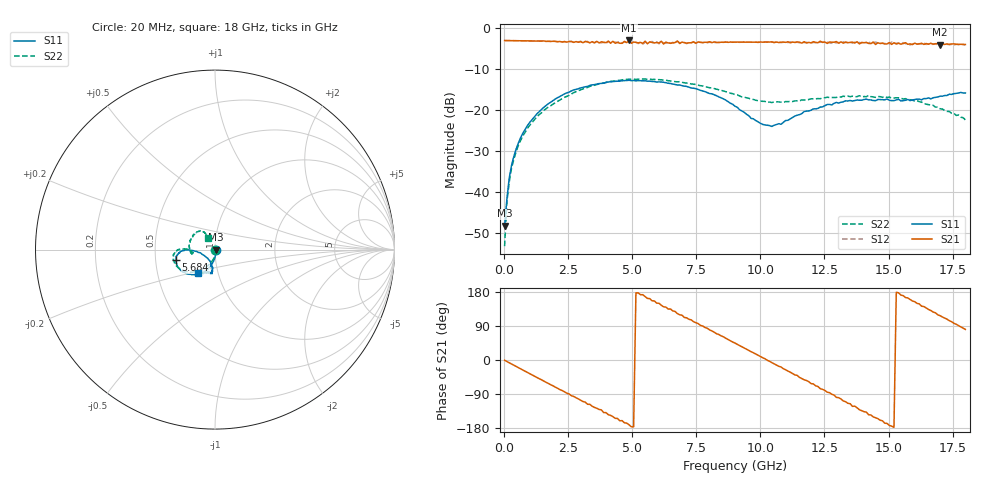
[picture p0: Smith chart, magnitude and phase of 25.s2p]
!Agilent Technologies,N5230A,US43500223,A.07.50.48
!Agilent N5230A: A.07.50.48
!Date: Monday, January 18, 2016 11:03:19
!Correction: S11(Full 2 Port(1,2))
!S21(Full 2 Port(1,2))
!S12(Full 2 Port(1,2))
!S22(Full 2 Port(1,2))
!S2P File: Measurements: S11, S21, S12, S22:
# Hz S  RI  R 50
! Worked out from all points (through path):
!   201 points, 20 MHz to 18 GHz, reference 50 ohm
!   highest |S21| = -3.01 dB at 4.875 GHz (marker M1); lowest = -4.0 dB at 17.01 GHz (marker M2)
!   group delay of S21, straight-line fit = 98.3 ps
!   lowest |S11| = -48.3 dB at 20 MHz (marker M3), VSWR 1.01, Z = 50.4 + j0.00489 ohm
!   |S11| at or under -10 dB: start of sweep to end of sweep
!   |S22| runs from -53.3 to -12.4 dB; largest |S21 - S12| = 0.065
!   S11 on the Smith chart (normalised r, x): 20 MHz: 1.01, +0.00; 5.684 GHz: 0.64, -0.08; 18 GHz: 0.80, -0.22
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2e7  0.00386 4.86e-05  0.7055 -0.00962  0.7061 -0.0107  0.00214 -0.000334
1.099e8  0.00412 -0.00706  0.7033 -0.0499  0.7034 -0.05  0.00412 -0.00636
1.998e8  0.00491 -0.0139  0.6984 -0.0896  0.6988 -0.0895  0.00385 -0.0125
6.493e8  -0.00112 -0.0462  0.6439 -0.2795  0.6433 -0.2806  -0.00368 -0.0426
1.9978e9  -0.0588 -0.1231  0.2175 -0.6546  0.2072 -0.6593  -0.0638 -0.1051
3.0766e9  -0.128 -0.1396  -0.2222 -0.6255  -0.2288 -0.631  -0.1305 -0.1255
3.7958e9  -0.1676 -0.1288  -0.4525 -0.5083  -0.4478 -0.4879  -0.1755 -0.1163
4.8746e9  -0.211 -0.0939  -0.6986 -0.1113  -0.6745 -0.1127  -0.2247 -0.0806
5.6837e9  -0.2176 -0.0579  -0.6479 0.211  -0.6343 0.2131  -0.2332 -0.0471
6.0433e9  -0.2165 -0.0415  -0.5677 0.3333  -0.5403 0.3488  -0.2324 -0.0335
7.3918e9  -0.1842 -0.00777  -0.1321 0.668  -0.132 0.6651  -0.2068 -0.00146
8.2009e9  -0.1534 -0.00105  0.1956 0.6509  0.201 0.6369  -0.1827 0.00422
9.01e9  -0.1107 -0.00873  0.4794 0.4756  0.4901 0.4605  -0.1542 0.00256
1.03585e10  -0.0457 -0.0454  0.6759 -0.0404  0.674 -0.0597  -0.1236 -0.0184
1.11676e10  -0.0249 -0.0737  0.5603 -0.3523  0.5644 -0.3771  -0.1249 -0.0253
1.20666e10  -0.0128 -0.1023  0.3091 -0.6094  0.2659 -0.6139  -0.1363 -0.0138
1.3505e10  -0.0169 -0.1296  -0.2876 -0.6061  -0.3268 -0.5873  -0.1414 0.0341
1.43141e10  -0.0204 -0.1312  -0.531 -0.3707  -0.5832 -0.3653  -0.1297 0.0661
1.50333e10  -0.0293 -0.1282  -0.6601 -0.0851  -0.637 -0.0762  -0.1123 0.09
1.57525e10  -0.0374 -0.129  -0.6102 0.1779  -0.6208 0.2207  -0.0874 0.103
1.70111e10  -0.0647 -0.1325  -0.2856 0.5601  -0.2654 0.5923  -0.0534 0.0887
1.8e10  -0.0928 -0.1323  0.1012 0.6241  0.1274 0.6074  -0.0401 0.0643
